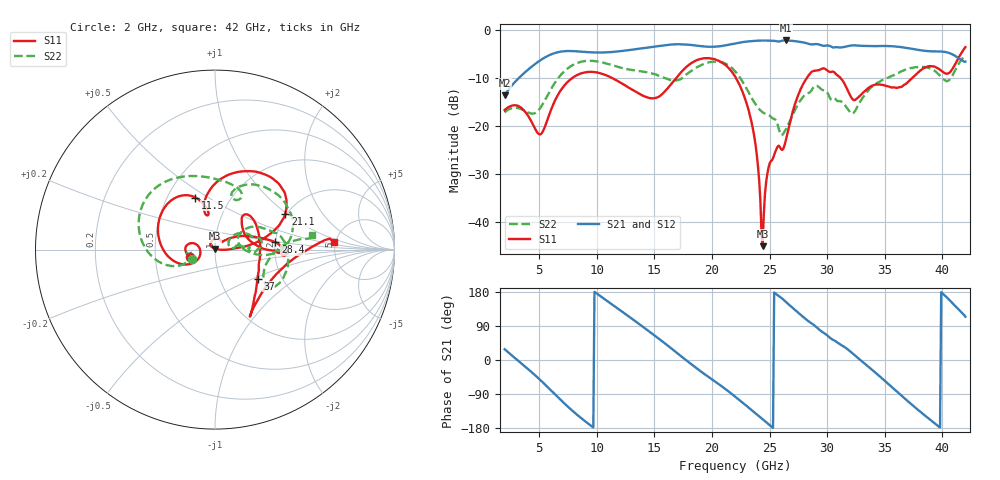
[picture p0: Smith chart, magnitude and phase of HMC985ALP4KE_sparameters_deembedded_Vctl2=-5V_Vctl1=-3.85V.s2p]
!s2p File: Measurements: S11, S21, S12, S22
# GHz S dB R 50.0
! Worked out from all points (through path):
!   401 points, 2 GHz to 42 GHz, reference 50 ohm
!   highest |S21| = -2.16 dB at 26.4 GHz (marker M1); lowest = -13.6 dB at 2 GHz (marker M2)
!   lowest |S11| = -45.0 dB at 24.4 GHz (marker M3), VSWR 1.01, Z = 49.9 + j0.551 ohm
!   |S11| at or under -10 dB: start of sweep to 7.86 GHz; 22.09 GHz to 28.23 GHz (6.136 GHz wide, 24.4 % of centre); 31.17 GHz to 37.37 GHz (6.201 GHz wide, 18.1 % of centre)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
!   |S22| runs from -21.9 to -5.3 dB; largest |S21 - S12| = 0.001
!   S11 on the Smith chart (normalised r, x): 2 GHz: 0.75, -0.06; 11.5 GHz: 0.69, +0.44; 21.1 GHz: 1.97, +0.97; 28.4 GHz: 2.00, +0.19; 37 GHz: 1.51, -0.53; 42 GHz: 4.86, +0.71
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2  -16.65 -163.9  -13.56 28.4  -13.56 28.4  -17.14 -158.9
5.1  -21.71 -171.4  -6.29 -52.8  -6.29 -52.8  -16.19 -159.0
6.3  -15.04 -152.0  -4.83 -88.3  -4.83 -88.3  -11.20 -161.3
8.7  -8.97 149.6  -4.50 -154.7  -4.50 -154.7  -6.56 151.5
11.5  -10.19 110.6  -4.53 142.8  -4.53 142.8  -7.42 105.6
13.6  -13.14 100.5  -3.91 96.7  -3.91 96.8  -8.50 76.6
15.4  -13.85 104.9  -3.33 55.9  -3.32 55.9  -9.50 63.4
17.9  -7.41 79.3  -3.04 -4.1  -3.04 -4.0  -9.03 71.7
21.1  -7.14 27.0  -3.21 -75.0  -3.21 -75.0  -6.92 15.8
22  -9.62 16.7  -2.78 -96.3  -2.78 -96.3  -8.55 0.6
23.5  -19.89 2.8  -2.28 -133.6  -2.28 -133.6  -14.32 -4.3
24.4  -44.96 101.9  -2.18 -156.3  -2.18 -156.2  -17.09 7.6
25  -27.79 130.0  -2.21 -171.5  -2.21 -171.5  -17.80 10.6
26.4  -23.04 44.3  -2.16 153.7  -2.16 153.8  -20.70 32.5
28.4  -9.40 7.1  -2.86 101.8  -2.86 101.8  -13.07 18.3
28.7  -8.61 1.9  -2.99 95.6  -2.99 95.6  -12.31 16.6
30.7  -8.98 -3.1  -3.58 50.2  -3.57 50.3  -14.29 2.8
32.4  -14.57 30.0  -3.18 12.3  -3.18 12.4  -16.92 26.8
35.4  -11.78 17.7  -3.33 -65.6  -3.33 -65.6  -9.79 18.9
37  -10.85 -34.3  -3.75 -108.6  -3.75 -108.6  -8.08 4.6
39.8  -8.26 -56.0  -4.45 -178.4  -4.45 -178.3  -9.49 -33.8
42  -3.55 3.5  -6.56 114.3  -6.57 114.3  -5.26 8.3
